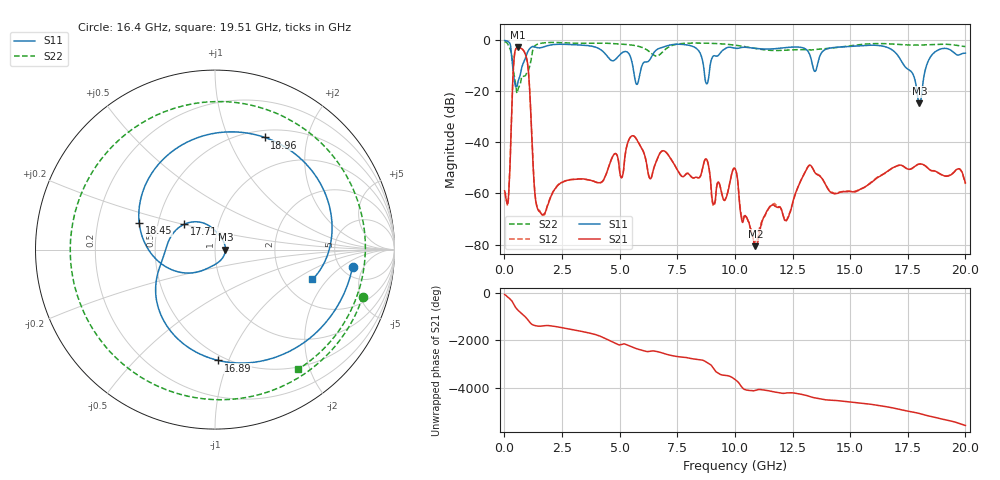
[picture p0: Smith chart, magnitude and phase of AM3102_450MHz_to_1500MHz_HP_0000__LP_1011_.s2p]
!Agilent Technologies,E8364B,MY43040894,A.07.50.67
!Agilent E8364B: A.07.50.67
!Date: Thursday, January 11, 2018 05:17:54
!Correction: S11(Full 2 Port(1,2))
!S21(Full 2 Port(1,2))
!S12(Full 2 Port(1,2))
!S22(Full 2 Port(1,2))
!S2P File: Measurements: S11, S21, S12, S22:
# Hz S  dB  R 50
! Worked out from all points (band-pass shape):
!   1601 points, 10 MHz to 20 GHz, reference 50 ohm
!   highest |S21| = -2.81 dB at 597.2 MHz (marker M1); lowest = -80.6 dB at 10.89 GHz (marker M2)
!   |S21| within 3 dB of the highest: 436.2 MHz to 923.9 MHz (487.8 MHz wide, 71.7 % of centre)
!   lowest |S11| = -24.7 dB at 18 GHz (marker M3), VSWR 1.12, Z = 56.2 + j0.0336 ohm
!   |S11| at or under -10 dB: 356.8 MHz to 775.1 MHz (418.4 MHz wide, 73.9 % of centre); 5.569 GHz to 5.966 GHz (397 MHz wide, 6.88 % of centre); 17.35 GHz to 18.31 GHz (955 MHz wide, 5.36 % of centre)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
!   |S22| runs from -20.7 to -0.5 dB; largest |S21 - S12| = 0.0012
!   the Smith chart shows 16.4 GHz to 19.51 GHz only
!   S11 on the Smith chart (normalised r, x): 16.4 GHz: 6.27, -3.05; 16.89 GHz: 0.46, -0.92; 17.71 GHz: 0.68, +0.20; 18.45 GHz: 0.39, +0.14; 18.96 GHz: 0.58, +1.37; 19.51 GHz: 2.86, -1.41
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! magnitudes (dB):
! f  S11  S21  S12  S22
! 10 MHz  0.0  -59.0  -59.5  -0.5
! 159.9 MHz  -0.5  -63.0  -63.8  -1.7
! 422.3 MHz  -15.2  -7.0  -7.0  -13.5
! 597.2 MHz  -16.0  -2.8  -2.8  -19.0
! 997 MHz  -4.8  -8.6  -8.6  -12.5
! 1.484 GHz  -2.9  -66.7  -66.3  -1.4
! 3.346 GHz  -1.9  -54.3  -54.4  -1.1
! 6.682 GHz  -3.3  -45.4  -45.4  -6.0
! 8.756 GHz  -16.9  -46.5  -46.5  -1.1
! 9.08 GHz  -6.1  -64.2  -64.9  -1.2
! 10.01 GHz  -3.1  -50.3  -50.2  -1.9
! 10.89 GHz  -3.1  -80.6  -78.7  -3.2
! 13.34 GHz  -8.6  -49.6  -49.6  -3.8
! 16.4 GHz  -2.2  -52.6  -52.6  -1.3
! 16.68 GHz  -3.0  -50.9  -51.0  -1.4
! 16.89 GHz  -4.2  -49.8  -49.8  -1.5
! 17.71 GHz  -13.1  -50.0  -50.1  -1.9
! 18 GHz  -24.7  -48.5  -48.4  -1.8
! 18.45 GHz  -7.0  -50.7  -50.7  -1.7
! 18.96 GHz  -3.3  -52.6  -52.7  -1.5
! 19.51 GHz  -4.9  -51.6  -51.6  -1.8
! 20 GHz  -5.0  -55.8  -56.3  -2.4
